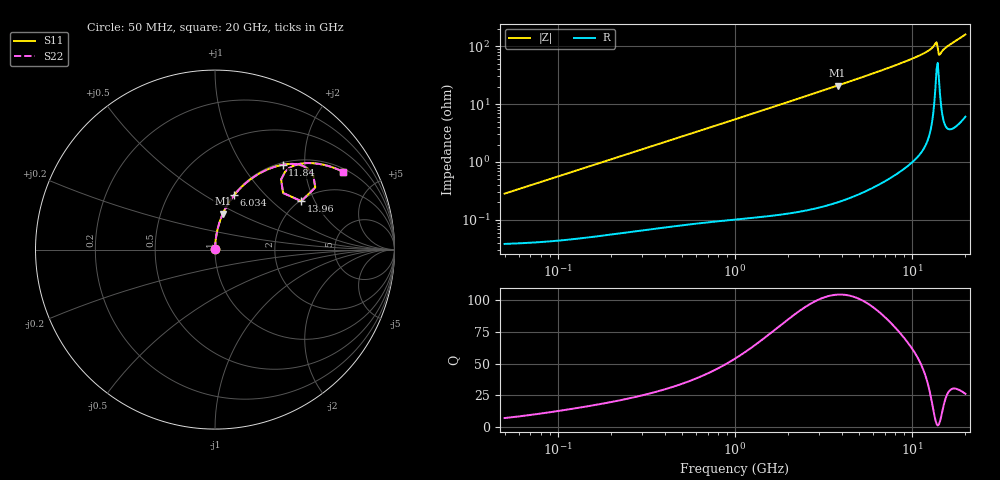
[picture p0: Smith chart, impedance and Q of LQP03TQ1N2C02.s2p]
!Murata Part Number: LQP03TQ1N2C02
!These Parameters are Measured in Series Mode Connection
!  o--[Z]--o
!Port1  Port2
!  o-------o
!Freq. Start=50[MHz] Stop=20[GHz], 401[Steps]
# Hz S RI R 50
!Freq.(Hz) S11(Real) S11(Imag) S21(Real) S21(Imag) S12(Real) S12(Imag) S22(Real) S22(Imag)
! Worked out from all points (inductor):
!   401 points, 50 MHz to 20 GHz, reference 50 ohm
!   read as one part in series: L = 896 pH near 51.52 MHz
!   highest Q = 104 at 3.793 GHz (marker M1), where L = 876 pH
!   S11 on the Smith chart (normalised r, x): 50 MHz: 1.00, +0.01; 6.034 GHz: 1.01, +0.68; 11.84 GHz: 1.04, +1.54; 13.96 GHz: 2.03, +1.58; 20 GHz: 1.12, +3.19
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5e7  0.000393 0.00282  0.9996 -0.00282  0.9996 -0.00282  0.000393 0.00282
1.364002e8  0.000541 0.00762  0.9995 -0.00762  0.9995 -0.00762  0.000541 0.00762
3.721004e8  0.00114 0.0205  0.9989 -0.0205  0.9989 -0.0205  0.00114 0.0205
1e9  0.00397 0.0543  0.996 -0.0543  0.996 -0.0543  0.00397 0.0543
1.714689e9  0.00983 0.0924  0.9902 -0.0924  0.9902 -0.0924  0.00983 0.0924
2.728004e9  0.0232 0.1455  0.9768 -0.1455  0.9768 -0.1455  0.0232 0.1455
3.792786e9  0.0435 0.1993  0.9565 -0.1993  0.9565 -0.1993  0.0435 0.1993
6.034176e9  0.1061 0.3027  0.8939 -0.3027  0.8939 -0.3027  0.1061 0.3027
7.442007e9  0.1577 0.3585  0.8423 -0.3585  0.8423 -0.3585  0.1577 0.3585
9.600142e9  0.2533 0.4273  0.7467 -0.4273  0.7467 -0.4273  0.2533 0.4273
1.183995e10  0.3767 0.4726  0.6233 -0.4726  0.6233 -0.4726  0.3767 0.4726
1.276073e10  0.447 0.4767  0.553 -0.4767  0.553 -0.4767  0.447 0.4767
1.314879e10  0.4895 0.4667  0.5105 -0.4667  0.5105 -0.4667  0.4895 0.4667
1.334722e10  0.517 0.4514  0.483 -0.4514  0.483 -0.4514  0.517 0.4514
1.354865e10  0.5473 0.4175  0.4527 -0.4175  0.4527 -0.4175  0.5473 0.4175
1.396067e10  0.4809 0.2698  0.5191 -0.2698  0.5191 -0.2698  0.4809 0.2698
1.417136e10  0.3792 0.3155  0.6208 -0.3155  0.6208 -0.3155  0.3792 0.3155
1.460232e10  0.39 0.4331  0.61 -0.4331  0.61 -0.4331  0.39 0.4331
1.504638e10  0.4371 0.4671  0.5629 -0.4671  0.5629 -0.4671  0.4371 0.4671
1.550395e10  0.4752 0.4783  0.5248 -0.4783  0.5248 -0.4783  0.4752 0.4783
1.721783e10  0.5799 0.4774  0.4201 -0.4774  0.4201 -0.4774  0.5799 0.4774
2e10  0.7105 0.4349  0.2895 -0.4349  0.2895 -0.4349  0.7105 0.4349
